FUNCTION FC 114 : VOID
TITLE =BLOCK START STOP CONVEYOR
AUTHOR : Esposito
FAMILY : EGAL_srl
NAME : CONVEYOR
VERSION : 0.1

BEGIN
NETWORK
TITLE =START SCRAP CONVEYOR
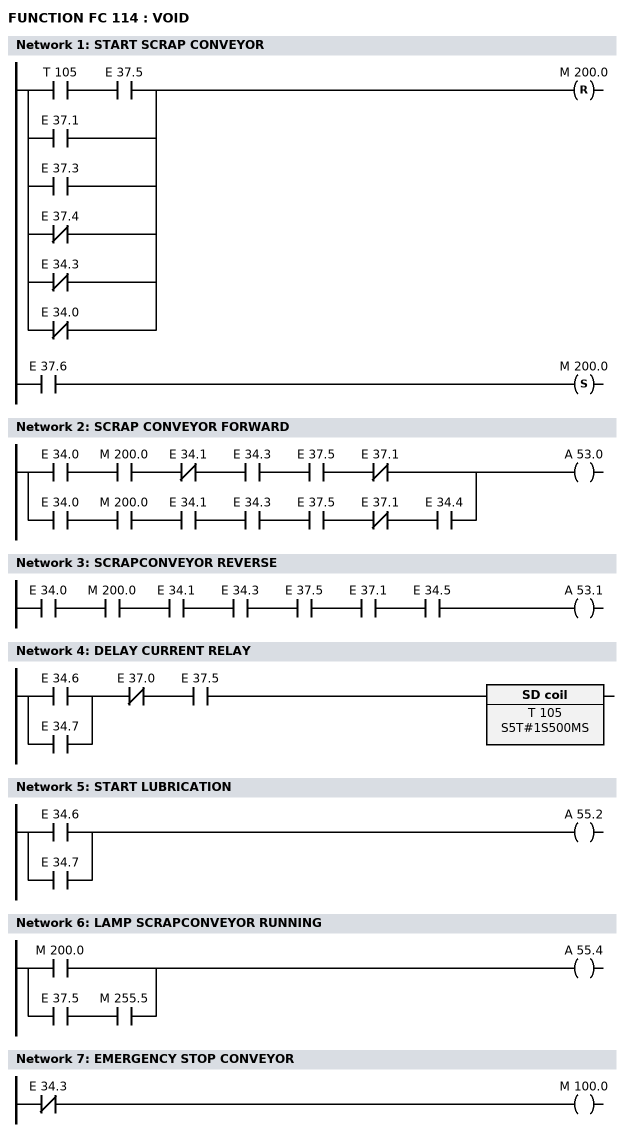
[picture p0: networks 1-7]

      U(    ;
      U     T    105;
      U     E     37.5;
      O     E     37.1;
      O     E     37.3;
      ON    E     37.4;
      ON    E     34.3;
      ON    E     34.0;
      )     ;
      R     M    200.0;
      U     E     37.6;
      S     M    200.0;
      NOP   0;
NETWORK
TITLE =SCRAP CONVEYOR FORWARD

      U     E     34.0;
      U     M    200.0;
      UN    E     34.1;
      U     E     34.3;
      U     E     37.5;
      UN    E     37.1;
      O     ;
      U     E     34.0;
      U     M    200.0;
      U     E     34.1;
      U     E     34.3;
      U     E     37.5;
      UN    E     37.1;
      U     E     34.4;
      =     A     53.0;
NETWORK
TITLE =SCRAPCONVEYOR REVERSE

      U     E     34.0;
      U     M    200.0;
      U     E     34.1;
      U     E     34.3;
      U     E     37.5;
      U     E     37.1;
      U     E     34.5;
      =     A     53.1;
NETWORK
TITLE =DELAY CURRENT RELAY

      U(    ;
      O     E     34.6;
      O     E     34.7;
      )     ;
      UN    E     37.0;
      U     E     37.5;
      L     S5T#1S500MS;
      SE    T    105;
      NOP   0;
      NOP   0;
      NOP   0;
      NOP   0;
NETWORK
TITLE =START LUBRICATION

      O     E     34.6;
      O     E     34.7;
      =     A     55.2;
NETWORK
TITLE =LAMP SCRAPCONVEYOR RUNNING

      O     M    200.0;
      O     ;
      U     E     37.5;
      U     M    255.5;
      =     A     55.4;
NETWORK
TITLE =EMERGENCY STOP CONVEYOR

      UN    E     34.3;
      =     M    100.0;
NETWORK
TITLE =FAULT PROXIMITY SWITCH CONVEYOR

      U(    ;
      O     E     34.6;
      O     E     34.7;
      )     ;
      UN    E     37.2;
      U     E     37.5;
      U     E     37.3;
      O(    ;
      U(    ;
      O     E     34.6;
      O     E     34.7;
      )     ;
      U     E     37.2;
      UN    E     37.5;
      U     E     37.3;
      L     S5T#5M;
      SE    T    106;
      NOP   0;
      NOP   0;
      NOP   0;
      U     T    106;
      )     ;
      =     M    100.1;
NETWORK
TITLE =ALARM MINIMUM LEVEL LUBRICATION
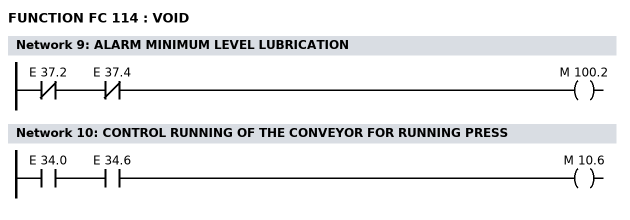
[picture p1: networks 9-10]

      UN    E     37.2;
      UN    E     37.4;
      =     M    100.2;
NETWORK
TITLE =CONTROL RUNNING OF THE CONVEYOR FOR RUNNING PRESS

      U     E     34.0;
      U     E     34.6;
      =     M     10.6;
END_FUNCTION

